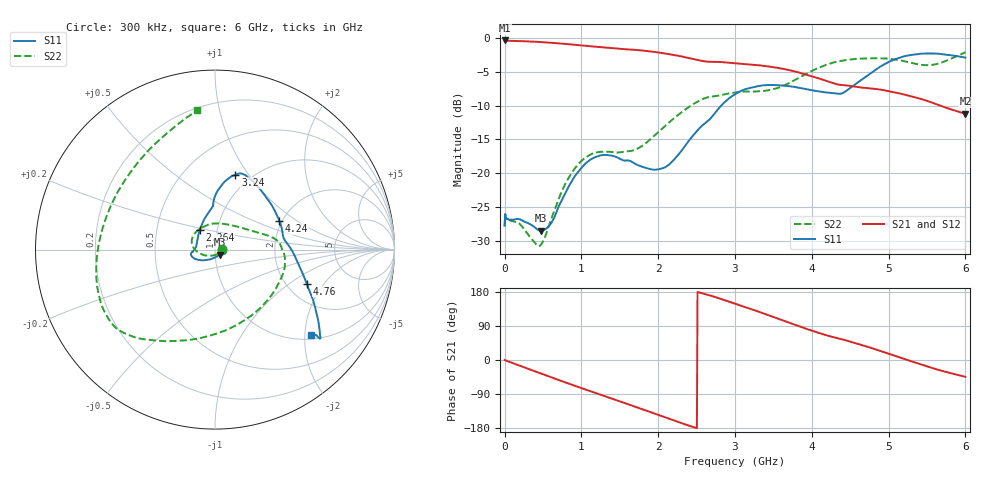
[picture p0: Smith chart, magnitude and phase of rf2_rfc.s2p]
!Agilent Technologies,M9375A,MY55441453,A.02.50.04
!Agilent M9375A: A.02.50.04
!Date: Monday, December 12, 2016 11:27:53
!Correction: S11(Full 2 Port(1,2))
!S21(Full 2 Port(1,2))
!S12(Full 2 Port(1,2))
!S22(Full 2 Port(1,2))
!S2P File: Measurements: S11, S21, S12, S22:
# Hz S  dB  R 50
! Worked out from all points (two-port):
!   751 points, 300 kHz to 6 GHz, reference 50 ohm
!   highest |S21| = -0.37 dB at 8.3 MHz (marker M1); lowest = -11.2 dB at 6 GHz (marker M2)
!   |S21| within 3 dB of the highest: start of sweep to 2.563 GHz
!   lowest |S11| = -28.5 dB at 472.3 MHz (marker M3), VSWR 1.08, Z = 52.6 - j2.88 ohm
!   |S11| at or under -10 dB: start of sweep to 2.82 GHz
!   |S22| runs from -30.8 to -2.1 dB; largest |S21 - S12| = 0.0012
!   S11 on the Smith chart (normalised r, x): 300 kHz: 1.09, -0.00; 2.264 GHz: 0.82, +0.18; 3.24 GHz: 0.85, +0.87; 4.24 GHz: 1.94, +0.73; 4.76 GHz: 2.55, -1.38; 6 GHz: 1.11, -2.16
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300000  -27.74 -2.2  -0.39 -0.1  -0.39 -0.1  -27.82 1.1
8299600  -26.04 3.4  -0.37 -0.6  -0.36 -0.6  -26.07 2.7
1.842908e8  -26.77 -3.2  -0.46 -14.1  -0.46 -14.1  -27.41 -12.4
4.722764e8  -28.49 -46.5  -0.60 -35.6  -0.60 -35.7  -30.57 -85.8
6.082696e8  -27.35 -88.2  -0.71 -45.8  -0.71 -45.8  -26.73 -132.4
7.762612e8  -23.27 -124.8  -0.87 -58.1  -0.86 -58.1  -21.88 -161.9
1.00025e9  -19.21 -148.6  -1.11 -74.1  -1.11 -74.2  -18.17 172.9
1.224239e9  -17.45 -163.3  -1.33 -89.9  -1.33 -89.9  -16.87 149.2
1.464227e9  -17.64 -173.1  -1.57 -106.7  -1.56 -106.8  -16.93 117.5
2.0002e9  -19.42 163.4  -2.14 -145.2  -2.14 -145.2  -13.93 35.6
2.264187e9  -17.24 128.4  -2.65 -164.0  -2.65 -164.1  -11.33 19.4
3.00015e9  -8.32 81.7  -3.74 148.7  -3.74 148.6  -8.07 -9.1
3.240138e9  -7.28 74.7  -3.98 132.4  -3.98 132.3  -7.93 -28.3
3.616119e9  -7.03 66.3  -4.55 104.8  -4.55 104.8  -7.13 -75.8
4.0001e9  -7.72 47.8  -5.66 77.4  -5.66 77.3  -4.87 -116.6
4.240088e9  -8.12 24.0  -6.54 62.3  -6.54 62.3  -3.78 -130.0
4.760062e9  -5.27 -20.4  -7.46 32.7  -7.45 32.7  -3.01 -144.9
5.00005e9  -3.56 -31.8  -7.86 16.5  -7.86 16.4  -3.07 -154.3
5.20004e9  -2.72 -37.2  -8.36 2.9  -8.36 2.8  -3.43 -169.2
5.432028e9  -2.32 -39.8  -9.05 -12.5  -9.05 -12.6  -3.99 163.3
5.728014e9  -2.45 -40.3  -10.24 -30.5  -10.23 -30.6  -3.47 122.0
6e9  -2.91 -41.4  -11.21 -44.3  -11.20 -44.3  -2.13 97.3
